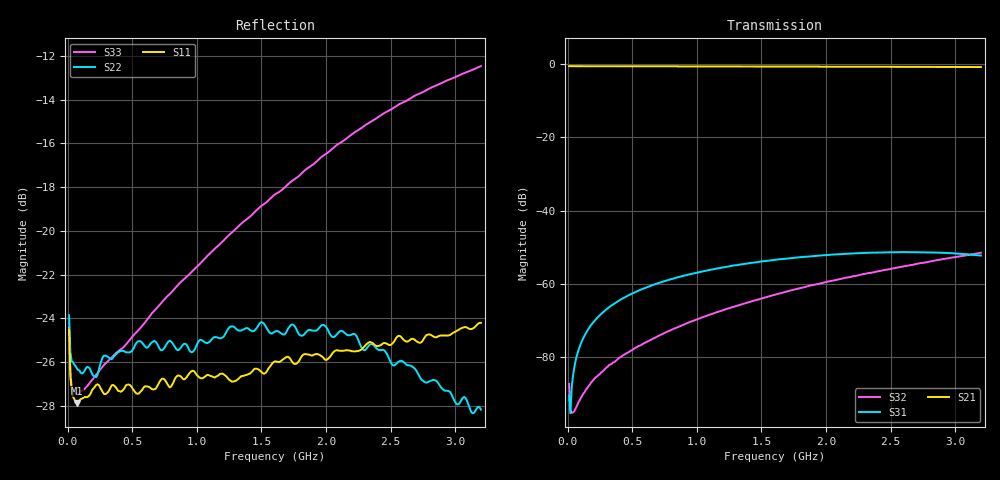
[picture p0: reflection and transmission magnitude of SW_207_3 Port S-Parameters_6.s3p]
! Created _Nov-02-2022_09-58-32
! Type : General
! Retest Level : 0
! Program : FASTESt Rev. 859
! DUT_TempC = 25.0
! Set_V1_Supply_V = 3.0
! V1_Supply_V = 3.0015
! V1_Supply_I = -6e-06
! Set_V2_Supply_V = 0.0
! V2_Supply_V = -0.001
! V2_Supply_I = -4e-06
! RunID = 6
! SN = 3
! Comment = SW-207_SB3_RFc-RF1_room
! Input_Power = 5.0
! Measurement_Comment = None
! Freq	S11db	S11deg	S12db	S12deg	S13db	S13deg	S21db	S21deg	S22db	S22deg	S23db	S23deg	S31db	S31deg	S32db	S32deg	S33db	S33deg
# Hz S dB R 50
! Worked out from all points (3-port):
!   320 points, 10 MHz to 3.2 GHz, reference 50 ohm
!   strongest paths, dB at 10 MHz, 810 MHz, 1.61 GHz, 2.41 GHz, 3.2 GHz:
!     S21: -0.6, -0.6, -0.7, -0.7, -0.8
!     S31: -90.5, -58.6, -53.4, -51.4, -52.2
!     S32: -87.3, -72.4, -62.8, -56.5, -51.5
!   lowest |S11| = -27.9 dB at 70 MHz (marker M1), VSWR 1.08, Z = 54.1 - j1.13 ohm
!   |S11| at or under -10 dB: start of sweep to end of sweep
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1e7  -24.50 -43.6  -0.58 1.2  -90.03 -124.9
     -0.58 1.2  -23.86 -39.9  -87.00 -112.8
     -90.46 -123.8  -87.26 -112.8  -24.41 -39.3
7e7  -27.86 -15.0  -0.59 -6.0  -79.55 79.9
     -0.59 -6.1  -26.28 -13.2  -93.15 -93.9
     -79.52 79.6  -93.26 -94.4  -27.43 -7.8
3.1e8  -27.38 -25.4  -0.60 -27.5  -66.58 63.0
       -0.61 -27.5  -25.76 -25.3  -82.61 -140.7
       -66.57 62.9  -82.49 -140.2  -25.96 -1.4
8.8e8  -26.67 -88.7  -0.63 -77.2  -57.90 18.4
       -0.63 -77.2  -25.30 -85.2  -71.39 149.7
       -57.87 18.4  -71.35 150.2  -22.31 -27.1
1.23e9  -26.66 -133.7  -0.65 -107.7  -55.30 -9.0
        -0.65 -107.7  -24.60 -125.8  -66.85 114.4
        -55.28 -9.1  -66.80 114.7  -20.30 -52.0
1.61e9  -25.96 -177.9  -0.68 -140.8  -53.41 -38.9
        -0.67 -140.8  -24.59 -166.8  -62.90 80.9
        -53.38 -38.9  -62.85 81.2  -18.32 -81.3
1.97e9  -25.75 140.2  -0.71 -172.0  -52.21 -67.6
        -0.70 -172.1  -24.30 155.8  -59.76 50.9
        -52.16 -67.8  -59.72 51.0  -16.60 -110.5
2.32e9  -25.15 107.2  -0.74 157.6  -51.49 -95.4
        -0.73 157.5  -25.33 118.7  -57.13 22.8
        -51.48 -95.3  -57.10 23.0  -15.11 -138.4
2.78e9  -24.76 65.4  -0.78 117.5  -51.37 -131.5
        -0.78 117.5  -26.94 70.4  -54.05 -11.6
        -51.35 -131.6  -54.03 -11.5  -13.56 -175.4
3.2e9  -24.20 26.2  -0.82 80.9  -52.25 -163.1
       -0.82 80.8  -28.17 19.3  -51.48 -42.0
       -52.23 -163.0  -51.45 -42.1  -12.48 150.3
